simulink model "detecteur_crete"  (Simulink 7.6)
settings: Solver=ode23tb  StartTime=0.0  StopTime=0.01  RelTol=1e-3
InitFcn:
  | clear all, clc
StopFcn:
  | % lecture du fichier binaire
  | load signaux.mat
  | 
  | % trace de la tension et du courant d’induit
  | plot(x(1,:),x(2,:),x(1,:),x(3,:),x(1,:),x(4,:))
  | title('détecteur de crête, sinus amorti et sinus du générateur')
  | grid
  | 
  | delete *.mat
libraries: fl_lib x8, nesl_utility x5, MaLibrairieElectrical_lib x2

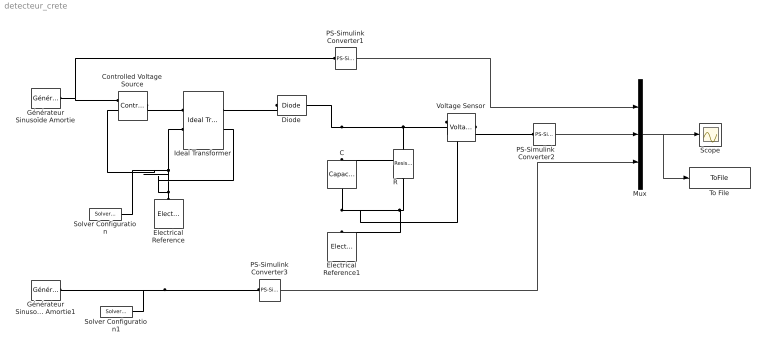
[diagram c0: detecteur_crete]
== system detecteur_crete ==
  C : fl_lib/Electrical/Electrical Elements/Capacitor  DialogController=NetworkEngine.DynNeDlgSource  SystemSampleTime=-1  c=220 nF  v0=0 V  r=1e-6 Ohm  g=0 1/Ohm  i_Log=off  v_Log=off  vc_Log=off  LocalVarNames=|i|v|vc  LocalVarDescs=|i|v|Internal variable for voltage across capacitor term  LocalVarLogging=[0 0 0]
  Controlled Voltage Source : fl_lib/Electrical/Electrical Sources/Controlled Voltage Source  DialogController=NetworkEngine.DynNeDlgSource  SystemSampleTime=-1  i_Log=off  v_Log=off  LocalVarNames=|i|v  LocalVarDescs=|i|v  LocalVarLogging=[0 0]
  Diode : fl_lib/Electrical/Electrical Elements/Diode  DialogController=NetworkEngine.DynNeDlgSource  SystemSampleTime=-1  Vf=0.6 V  Ron=0.3 Ohm  Goff=1e-8 1/Ohm  i_Log=off  v_Log=off  LocalVarNames=|i|v  LocalVarDescs=|i|v  LocalVarLogging=[0 0]
  Electrical Reference : fl_lib/Electrical/Electrical Elements/Electrical Reference  DialogController=NetworkEngine.DynNeDlgSource  SystemSampleTime=-1  i_Log=off  LocalVarNames=|i  LocalVarDescs=|i  LocalVarLogging=0
  Electrical Reference1 : fl_lib/Electrical/Electrical Elements/Electrical Reference  DialogController=NetworkEngine.DynNeDlgSource  SystemSampleTime=-1  i_Log=off  LocalVarNames=|i  LocalVarDescs=|i  LocalVarLogging=0
  Générateur Sinusoïde Amortie : MaLibrairieElectrical_lib/Générateur Sinusoïde Amortie  DialogController=NetworkEngine.DynNeDlgSource  SystemSampleTime=-1  biais=0  w=6.2832*1e3/4 1/s  Amp=1  phi=0 rad  a=0  LocalVarLogging=[]
  Générateur Sinusoïde Amortie1 : MaLibrairieElectrical_lib/Générateur Sinusoïde Amortie  DialogController=NetworkEngine.DynNeDlgSource  SystemSampleTime=-1  biais=0  w=6.2832*1e3/4 1/s  Amp=1  phi=0 rad  a=200  LocalVarLogging=[]
  Ideal Transformer : fl_lib/Electrical/Electrical Elements/Ideal Transformer  DialogController=NetworkEngine.DynNeDlgSource  SystemSampleTime=-1  n=0.5  i1_Log=off  v1_Log=off  i2_Log=off  v2_Log=off  LocalVarNames=|i1|v1|i2|v2  LocalVarDescs=|i1|v1|i2|v2  LocalVarLogging=[0 0 0 0]
  Mux : Mux  Inputs=3
  PS-Simulink Converter1 : nesl_utility/PS-Simulink Converter  DialogController=NetworkEngine.DynNeUtilDlgSource  SystemSampleTime=-1  PhysicalDomain=network_engine_domain  LeftPortType=input  RightPortType=output  SubClassName=ps_output  Unit=1  AffineConversion=off
  PS-Simulink Converter2 : nesl_utility/PS-Simulink Converter  DialogController=NetworkEngine.DynNeUtilDlgSource  SystemSampleTime=-1  PhysicalDomain=network_engine_domain  LeftPortType=input  RightPortType=output  SubClassName=ps_output  Unit=1  AffineConversion=off
  PS-Simulink Converter3 : nesl_utility/PS-Simulink Converter  DialogController=NetworkEngine.DynNeUtilDlgSource  SystemSampleTime=-1  PhysicalDomain=network_engine_domain  LeftPortType=input  RightPortType=output  SubClassName=ps_output  Unit=1  AffineConversion=off
  R : fl_lib/Electrical/Electrical Elements/Resistor  DialogController=NetworkEngine.DynNeDlgSource  SystemSampleTime=-1  R=470 kOhm  i_Log=off  v_Log=off  LocalVarNames=|i|v  LocalVarDescs=|i|v  LocalVarLogging=[0 0]
  Scope : Scope
  Solver Configuration : nesl_utility/Solver Configuration  DialogController=NetworkEngine.DynNeUtilDlgSource  SystemSampleTime=-1  PhysicalDomain=network_engine_domain  LeftPortType=input  RightPortType=generic  SubClassName=solver  Accelerate=off  Profile=off  ResidualTolerance=1e-9  MaxNonlinIter=3  MaxModeIter=2  DoFixedCost=off  UseLocalSampling=off  DoDC=off  LinearAlgebra=Sparse  LocalSolverSampleTime=.001  LocalSolverChoice=NE_BACKWARD_EULER_ADVANCER  UseLocalSolver=off
  Solver Configuration1 : nesl_utility/Solver Configuration  DialogController=NetworkEngine.DynNeUtilDlgSource  SystemSampleTime=-1  PhysicalDomain=network_engine_domain  LeftPortType=input  RightPortType=generic  SubClassName=solver  Accelerate=off  Profile=off  ResidualTolerance=1e-9  MaxNonlinIter=3  MaxModeIter=2  DoFixedCost=off  UseLocalSampling=off  DoDC=off  LinearAlgebra=Sparse  LocalSolverSampleTime=.001  LocalSolverChoice=NE_BACKWARD_EULER_ADVANCER  UseLocalSolver=off
  To File : ToFile  Filename=signaux  MatrixName=x
  Voltage Sensor : fl_lib/Electrical/Electrical Sensors/Voltage Sensor  DialogController=NetworkEngine.DynNeDlgSource  SystemSampleTime=-1  i1_Log=off  v1_Log=off  LocalVarNames=|i1|v1  LocalVarDescs=|i1|v1  LocalVarLogging=[0 0]
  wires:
  PS-Simulink Converter2/1 -> Mux/2
  PS-Simulink Converter1/1 -> Mux/1
  Mux/1 -> Scope/1, To File/1
  PS-Simulink Converter3/1 -> Mux/3
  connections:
  Générateur Sinusoïde Amortie/RConn1 -- Controlled Voltage Source/RConn1 -- PS-Simulink Converter1/LConn1
  Controlled Voltage Source/LConn1 -- Ideal Transformer/LConn1
  Voltage Sensor/RConn1 -- PS-Simulink Converter2/LConn1
  Diode/RConn1 -- C/RConn1 -- Voltage Sensor/LConn1 -- R/RConn1
  Diode/LConn1 -- Ideal Transformer/RConn1
  PS-Simulink Converter3/LConn1 -- Générateur Sinusoïde Amortie1/RConn1 -- Solver Configuration1/RConn1
  Electrical Reference/LConn1 -- Ideal Transformer/LConn2 -- Controlled Voltage Source/RConn2 -- Solver Configuration/RConn1 -- Ideal Transformer/RConn2
  C/LConn1 -- Electrical Reference1/LConn1 -- R/LConn1 -- Voltage Sensor/RConn2
